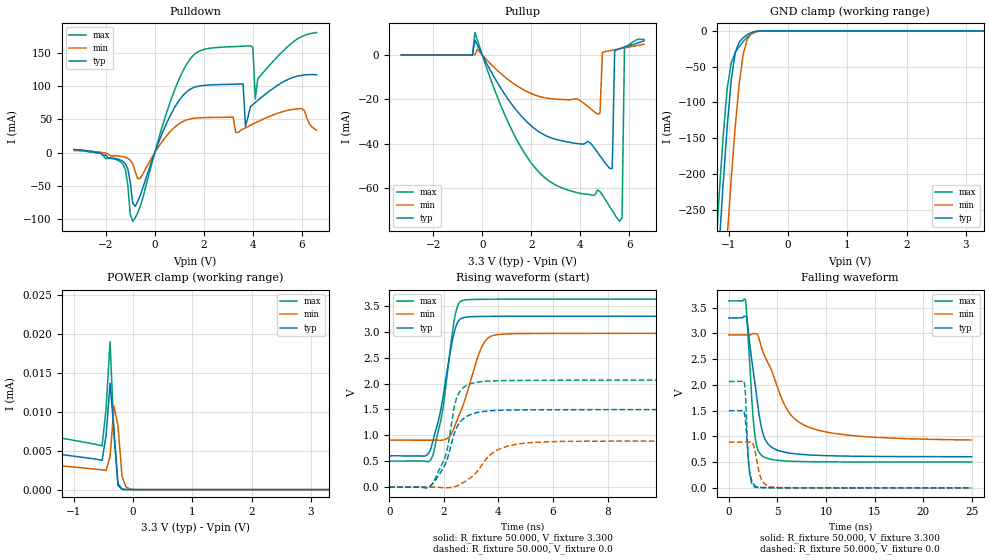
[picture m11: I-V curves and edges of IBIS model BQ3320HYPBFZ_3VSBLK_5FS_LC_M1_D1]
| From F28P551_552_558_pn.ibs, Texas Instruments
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|   Model BQ3320HYPBFZ_3VSBLK_5FS_LC_M1_D1
[Model] BQ3320HYPBFZ_3VSBLK_5FS_LC_M1_D1
Model_type I/O
Polarity   Non-Inverting
Enable   Active-Low
Vinl =  0.990V
Vinh =  2.310V
Vmeas =  1.650V
C_comp   3.470pF   3.136pF   3.588pF
[Model Spec]
Vinh   2.310V   2.079V   2.541V
Vinl   0.990V   0.891V   1.089V
Vmeas   1.650V   1.485V   1.815V
[Temperature Range]   25.000   0.155k   -40.000
[Voltage Range]   3.300V   2.970V   3.630V
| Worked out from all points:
|   slope of the pulldown table from 0 to 0.495 V, typ, clamps not added: 10.9 ohm
|   slope of the pullup table from 0 to 0.495 V, typ, clamps not added: 48.7 ohm
|   GND clamp passes 1 mA (typ) near -0.56 V on its own axis
|   rising waveform, R_fixture 50.000, V_fixture 3.300: 20-80 % time 559ps typ, 769ps min, 501ps max; typ from 0.605 V to 3.3 V
|   rising waveform, R_fixture 50.000, V_fixture 0.0: 20-80 % time 617ps typ, 974ps min, 526ps max; typ from 0 V to 1.5 V
|   falling waveform, R_fixture 50.000, V_fixture 3.300: 20-80 % time 1.21ns typ, 3.11ns min, 663ps max; typ from 3.3 V to 0.605 V
|   falling waveform, R_fixture 50.000, V_fixture 0.0: 20-80 % time 392ps typ, 623ps min, 307ps max; typ from 1.5 V to 0 V
[Pulldown]
|Voltage   I(typ)   I(min)   I(max)
-3.3V     4.877mA    3.346mA    4.741mA
-1.3V     -13.05mA   -6.062mA   -17.42mA
-900mV    -76.2mA    -16.7mA    -103.3mA
-600mV    -64.99mA   -38.74mA   -81.7mA
700mV     60.75mA    34.43mA    83.66mA
1.6V      98.27mA    51.81mA    147.5mA
3.6V      103.6mA    35.59mA    160.4mA
3.7V      39.88mA    37.53mA    160.6mA
4V        72.48mA    43.12mA    158.8mA
4.1V      75.66mA    44.92mA    80.91mA
6V        116.5mA    66.27mA    175mA
6.6V      117.2mA    33.89mA    180.9mA
[Pullup]
|Voltage   I(typ)   I(min)   I(max)
-3.3V     91.12nA    732.4nA    262.6pA
-300mV    6.771mA    40uA       10.12mA
2.1V      -32.9mA    -17.84mA   -50.16mA
4.7V      -43.94mA   -26.62mA   -60.94mA
4.8V      -45.49mA   -26.33mA   -61.57mA
4.9V      -46.98mA   1.13mA     -63.18mA
5.3V      -51.24mA   2.168mA    -70.17mA
5.4V      1.932mA    2.379mA    -71.96mA
5.6V      2.89mA     2.796mA    -75.03mA
5.7V      3.22mA     3.002mA    -73.63mA
5.8V      3.551mA    3.206mA    3.6mA
6.6V      6.408mA    4.882mA    7.034mA
[GND_clamp]
|Voltage   I(typ)   I(min)   I(max)
-3.3V     -3.505A    -3.628A    -3.476A
-1.223V   -386.4mA   -550.8mA   -315.4mA
-1.156V   -296.3mA   -460mA     -226.1mA
-1.089V   -210.5mA   -371.5mA   -144.6mA
-1.022V   -132.4mA   -286.5mA   -79.77mA
-955mV    -68.78mA   -206.3mA   -44.76mA
-888mV    -30.47mA   -133.9mA   -30.31mA
-821mV    -15.84mA   -73.99mA   -22.01mA
-754mV    -9.591mA   -32.92mA   -15.01mA
-687mV    -5.432mA   -12.28mA   -9.043mA
-620mV    -2.525mA   -4.288mA   -4.466mA
3.3V      0A         0A         0A
[POWER_clamp]
|Voltage   I(typ)   I(min)   I(max)
-3.3V     514.6uA    72.31mA    9.489uA
-3.266V   143.9uA    52.63mA    9.442uA
-3.132V   7.182uA    5.855mA    9.258uA
-2.931V   6.231uA    34.42uA    8.983uA
-2.864V   6.164uA    9.16uA     8.891uA
-2.73V    6.03uA     4.29uA     8.707uA
-519mV    3.757uA    2.535uA    5.612uA
-385mV    13.66uA    4.234uA    18.99uA
-318mV    7.479uA    10.7uA     6.925uA
-251mV    757.2nA    8.165uA    518.6nA
-184mV    65.2nA     1.742uA    33.01nA
3.3V      0A         0A         0A
[Ramp]
| variable   typ   min   max
dV/dt_r   0.899/0.618n   0.533/0.974n   1.240/0.527n
dV/dt_f   1.617/1.213n   1.225/3.111n   1.876/0.663n
R_load = 50.000
[Rising Waveform]
R_fixture= 50.000
V_fixture= 3.300
V_fixture_min= 2.970
V_fixture_max= 3.630
|time   V(typ)   V(min)   V(max)
0s        604.5mV    907.6mV    502.5mV
1.305ns   601.3mV    908.1mV    500.8mV
1.57ns    826.9mV    908.1mV    574.5mV
1.969ns   1.735V     909.3mV    1.518V
2.408ns   3.043V     1.185V     3.299V
2.537ns   3.209V     1.36V      3.536V
2.712ns   3.271V     1.59V      3.608V
3.382ns   3.296V     2.697V     3.627V
3.958ns   3.298V     2.943V     3.628V
25ns      3.3V       2.97V      3.63V
[Rising Waveform]
R_fixture= 50.000
V_fixture= 0.0
V_fixture_min= 0.0
V_fixture_max= 0.0
|time   V(typ)   V(min)   V(max)
0s        2.237uV    2.235uV    1.89uV
1.539ns   39.26mV    961.7uV    33.52mV
2.077ns   469.5mV    -12.54mV   628.9mV
2.376ns   1.021V     4.737mV    1.528V
2.508ns   1.188V     28.46mV    1.769V
2.786ns   1.348V     111.1mV    1.948V
3.236ns   1.443V     311.9mV    2.029V
4ns       1.483V     725.6mV    2.055V
5.52ns    1.494V     870.4mV    2.063V
25ns      1.498V     888.2mV    2.066V
[Falling Waveform]
R_fixture= 50.000
V_fixture= 3.300
V_fixture_min= 2.970
V_fixture_max= 3.630
|time   V(typ)   V(min)   V(max)
0s        3.3V       2.97V      3.63V
1.718ns   3.331V     2.97V      3.647V
1.876ns   3.264V     2.97V      3.249V
2.398ns   2.424V     2.99V      1.62V
2.631ns   2.119V     2.997V     1.106V
2.96ns    1.632V     2.978V     754.6mV
3.511ns   1.053V     2.646V     611.9mV
5.918ns   686.4mV    1.547V     521.6mV
8.008ns   642.4mV    1.196V     509.2mV
25ns      605.1mV    929.1mV    502.6mV
[Falling Waveform]
R_fixture= 50.000
V_fixture= 0.0
V_fixture_min= 0.0
V_fixture_max= 0.0
|time   V(typ)   V(min)   V(max)
0s        1.498V     888.2mV    2.066V
1.579ns   1.468V     888.1mV    2.056V
1.714ns   1.311V     888.1mV    1.807V
1.944ns   717.4mV    888mV      754.5mV
2.076ns   422.3mV    888mV      385.4mV
2.32ns    163.8mV    894.7mV    112.5mV
2.639ns   49.74mV    765.3mV    17.84mV
3.33ns    6.809mV    176.7mV    4.523mV
4.387ns   2.431mV    17.36mV    2.167mV
25ns      13.26uV    52.33uV    22.28uV
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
